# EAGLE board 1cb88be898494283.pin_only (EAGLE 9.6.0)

Size 43.18 x 43.18 mm. Coordinates in mm from the lower left corner, seen from the top.
Outline: 43.18,0 0,0 0,43.18 43.18,43.18 43.18,0
Copper layers (1+2*15+16): Top 0.035mm / dielectric 1.5mm / Route2 0.035mm / dielectric 0.15mm / Route15 0.035mm / dielectric 0.2mm / Bottom 0.035mm
Design rules "SparkFun-4-layer-MicroMod *": minimum track width 4mil, minimum drill 0.2mm, track to track 4mil, track to pad 4mil, pad to pad 4mil, via to via 4mil, smd to smd 4mil, copper to edge 6mil, drill to drill 6mil, minimum pad ring 6mil, minimum via ring 6mil, stop-mask expansion 4mil, vias tented up to drill 25mil, thermal gap 10mil
Net classes: 1 power: width 0.178 mm; 2 3.3V: width 0.508 mm; 3 RF: width 0.35 mm, clearance 0.203 mm

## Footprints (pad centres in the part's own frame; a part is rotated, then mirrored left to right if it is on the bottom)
ML414H_IV01E = smd 1 x 1: + 2.022,2.032 | smd 4.2 x 1.7: - 0.6,-1.85
0402 = smd 0.85 x 0.9: 1 -0.58,0; 2 0.58,0
0603 = smd 1.1 x 1: 1 -0.85,0; 2 0.85,0
LED-0603 = smd 1 x 1: A -0.877,0; C 0.877,0
SOD-323 = smd 0.63 x 0.83: A 1.15,0; C -1.15,0
SOT886 = smd 0.61 x 0.25: 1 -0.405,0.5 | smd 0.56 x 0.25: 2 -0.43,0; 3 -0.43,-0.5; 4 0.43,-0.5; 5 0.43,0; 6 0.43,0.5
SMA-EDGE = smd 1.5 x 4: GND@0 -2.54,0; GND@1 2.54,0; SIG 0,0 | smd 1.5 x 4 bottom: GND@2 -2.54,0; GND@3 2.54,0
0402_MURATA = smd 0.4 x 0.7: P1 -0.4,0; P2 0.4,0
SMT-JUMPER_2_NC_TRACE_SILK = smd 0.66 x 1.27: 1 -0.521,0; 2 0.521,0
1X06_NO_SILK = drill 1.016 pad 1.88: 1 0,0; 2 2.54,0; 3 5.08,0; 4 7.62,0; 5 10.16,0; 6 12.7,0
JST04_1MM_RA = smd 0.6 x 1.35: 1 -1.5,0; 2 -0.5,0; 3 0.5,0; 4 1.5,0 | smd 1.2 x 2: NC1 2.8,-3.675; NC2 -2.8,-3.675
1X04_NO_SILK = drill 1.016 pad 1.88: 1 0,0; 2 2.54,0; 3 5.08,0; 4 7.62,0
USB-C-16P-2LAYER-PADS = smd 0.3 x 1: A5 -1.25,-0.34; A6 -0.25,-0.34; A7 0.25,-0.34; A8 1.25,-0.34; B5 1.75,-0.34; B6 0.75,-0.34; B7 -0.75,-0.34; B8 -1.75,-0.34 | smd 0.6 x 1: GND -3.225,-0.34; GND2 3.225,-0.34; VBUS1 -2.45,-0.34; VBUS2 2.45,-0.34 | drill 0.4 pad 0.6 long: SHLD1 -4.318,-0.915; SHLD2 4.318,-0.915; SHLD3 -4.318,-5.095; SHLD4 4.318,-5.095 | hole 0.65: -2.89,-1.445; 2.89,-1.445
1X09_NO_SILK = drill 1.016 pad 1.88: 1 0,0; 2 2.54,0; 3 5.08,0; 4 7.62,0; 5 10.16,0; 6 12.7,0; 7 15.24,0; 8 17.78,0; 9 20.32,0
SMT-JUMPER_3_2-NC_TRACE_SILK = smd 0.66 x 1.27: 1 -1.041,0; 2 0,0; 3 1.041,0
MICRO-FIDUCIAL = smd 0.635 x 0.635: 1 0,0
STAND-OFF = hole 3.302: 0,0
SMT-JUMPER_2_NO_SILK = smd 0.635 x 1.27: 1 -0.406,0; 2 0.406,0
SOT23-5 = smd 0.55 x 1.2: 1 -0.95,-1.3; 2 0,-1.3; 3 0.95,-1.3; 4 0.95,1.3; 5 -0.95,1.3
ZED-F9P = smd 0.85 x 1.52: 1 -7.15,-7.45; 2 -6.05,-7.45; 3 -4.95,-7.45; 4 -3.85,-7.45; 5 -2.75,-7.45; 6 -1.65,-7.45; 7 -0.55,-7.45; 8 0.55,-7.45; 9 1.65,-7.45; 10 2.75,-7.45; 11 3.85,-7.45; 12 4.95,-7.45; 13 6.05,-7.45; 14 7.15,-7.45; 28 7.15,7.45; 29 6.05,7.45; 30 4.95,7.45; 31 3.85,7.45; 32 2.75,7.45; 33 1.65,7.45; 34 0.55,7.45; 35 -0.55,7.45; 36 -1.65,7.45; 37 -2.75,7.45; 38 -3.85,7.45; 39 -4.95,7.45; 40 -6.05,7.45; 41 -7.15,7.45 | smd 1.52 x 0.85: 15 9.95,-6.6; 16 9.95,-5.5; 17 9.95,-4.4; 18 9.95,-3.3; 19 9.95,-2.2; 20 9.95,-1.1; 21 9.95,0; 22 9.95,1.1; 23 9.95,2.2; 24 9.95,3.3; 25 9.95,4.4; 26 9.95,5.5; 27 9.95,6.6; 42 -9.95,6.6; 43 -9.95,5.5; 44 -9.95,4.4; 45 -9.95,3.3; 46 -9.95,2.2; 47 -9.95,1.1; 48 -9.95,0; 49 -9.95,-1.1; 50 -9.95,-2.2; 51 -9.95,-3.3; 52 -9.95,-4.4; 53 -9.95,-5.5; 54 -9.95,-6.6 | smd 1.1 x 1.1: 55 -1.05,-1.05; 56 -3.15,-1.05; 57 -5.25,-1.05; 58 -7.35,-1.05; 59 -1.05,-3.1; 60 -3.15,-3.1; 61 -5.25,-3.1; 62 -7.35,-3.1; 63 -1.05,-5.15; 64 -3.15,-5.15; 65 -5.25,-5.15; 66 -7.35,-5.15; 67 -1.05,5.15; 68 -3.15,5.15; 69 -5.25,5.15; 70 -7.35,5.15; 71 -1.05,3.1; 72 -3.15,3.1; 73 -5.25,3.1; 74 -7.35,3.1; 75 -1.05,1.05; 76 -3.15,1.05; 77 -5.25,1.05; 78 -7.35,1.05; 79 1.05,1.05; 80 3.15,1.05; 81 5.25,1.05; 82 7.35,1.05; 83 1.05,3.1; 84 3.15,3.1; 85 5.25,3.1; 86 7.35,3.1; 87 1.05,5.15; 88 3.15,5.15; 89 5.25,5.15; 90 7.35,5.15; 91 1.05,-5.15; 92 3.15,-5.15; 93 5.25,-5.15; 94 7.35,-5.15; 95 1.05,-3.1; 96 3.15,-3.1; 97 5.25,-3.1; 98 7.35,-3.1; 99 1.05,-1.05; 100 3.15,-1.05; 101 5.25,-1.05; 102 7.35,-1.05

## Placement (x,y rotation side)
B1  6.8MM_COIN_CELL  [ML414H_IV01E]  11.43,29.21 180 top
C1  47pF  [0402]  35.05,23.24 90 top
C2  1.0uF  [0603]  13.97,19.81 180 top
C3  1.0uF  [0603]  11.05,16.76 270 top
C4  1.0uF  [0603]  15.24,26.67 0 top
C5  0.1uF  [0603]  15.88,24.13 270 top
C6  1.0uF  [0603]  9.53,24.13 90 top
C7  0.1uF  [0603]  13.97,18.29 0 top
D1  Yellow  [LED-0603]  37.47,30.48 270 top
D2  0.5A/40V/420mV  [SOD-323]  13.97,21.34 0 top
D3  GREEN  [LED-0603]  39.37,30.48 270 top
D4  BLUE  [LED-0603]  41.27,30.48 270 top
D6  PRTR5V0U2F  [SOT886]  10.92,13.08 0 top
E1  SMA  [SMA-EDGE]  41.02,19.43 270 top
E2  SMA  [SMA-EDGE]  41.02,10.03 270 top
FB1  120NH  [0402_MURATA]  35.05,16.13 90 top
FENCE  [SMT-JUMPER_2_NC_TRACE_SILK]  41.27,31.75 270 bottom
FRAME2  FRAME-LEDGER  [CREATIVE_COMMONS]  not placed on the board
J1  Radio  [1X06_NO_SILK]  1.27,34.29 270 top
J2  Qwiic Right Angle  [JST04_1MM_RA]  8.89,5.08 0 top
J3  PTH  [1X04_NO_SILK]  13.97,1.27 0 top
J4  Qwiic Right Angle  [JST04_1MM_RA]  8.89,38.1 180 top
J5  [USB-C-16P-2LAYER-PADS]  6.35,12.7 270 top
J6  [1X06_NO_SILK]  24.13,1.27 0 top
J7  [1X09_NO_SILK]  34.29,41.91 180 top
JP5  [SMT-JUMPER_3_2-NC_TRACE_SILK]  11.43,8.89 0 top
JP21  FIDUCIALUFIDUCIAL  [MICRO-FIDUCIAL]  42.55,42.55 90 top
JP31  STAND-OFF  [STAND-OFF]  2.54,2.54 90 top
JP41  STAND-OFF  [STAND-OFF]  2.54,40.64 90 top
JP61  FIDUCIALUFIDUCIAL  [MICRO-FIDUCIAL]  0.64,0.64 90 top
JP71  FIDUCIALUFIDUCIAL  [MICRO-FIDUCIAL]  42.55,42.55 270 bottom
JP81  FIDUCIALUFIDUCIAL  [MICRO-FIDUCIAL]  0.64,0.64 270 bottom
JP91  STAND-OFF  [STAND-OFF]  40.64,2.54 90 top
JP101  STAND-OFF  [STAND-OFF]  40.64,40.64 90 top
LED2  RED  [LED-0603]  35.56,30.48 270 top
LOGO1  OSHW-LOGOMINI  [OSHW-LOGO-MINI]  2.54,5.59 0 bottom
LOGO2  SFE_LOGO_NAME_FLAME.1_INCH  [SFE_LOGO_NAME_FLAME_.1]  21.59,25.4 0 bottom
PPS  [SMT-JUMPER_2_NC_TRACE_SILK]  33.02,7.62 90 top
PPS_LED  [SMT-JUMPER_2_NC_TRACE_SILK]  36.2,31.75 270 bottom
PWR  [SMT-JUMPER_2_NC_TRACE_SILK]  33.78,31.75 270 bottom
R1  1k  [0603]  35.56,34.29 90 top
R2  33  [0603]  21.46,7.62 270 top
R3  33  [0603]  18.41,7.62 270 top
R4  33  [0603]  22.99,7.62 270 top
R5  1k  [0603]  10.92,20.32 90 top
R6  33  [0603]  19.94,7.62 270 top
R7  2.2k  [0603]  13.97,8.89 90 top
R8  2.2k  [0603]  8.89,8.89 90 top
R9  27  [0603]  13.97,13.72 0 top
R10  27  [0603]  13.97,15.24 0 top
R11  1k  [0603]  37.47,34.29 90 top
R12  1k  [0603]  39.37,34.29 90 top
R13  1k  [0603]  41.27,34.29 90 top
R14  33  [0603]  35.05,19.81 90 top
R15  100k  [0603]  13.97,16.76 0 top
R16  5.1k  [0603]  3.17,6.99 0 top
R17  5.1k  [0603]  3.17,18.41 0 top
R18  33  [0603]  29.72,7.62 270 top
R19  33  [0603]  26.67,7.62 270 top
R20  33  [0603]  28.19,7.62 270 top
R21  33  [0603]  31.24,7.62 270 top
R22  33  [0603]  20.45,35.56 90 top
R23  33  [0603]  18.92,35.56 90 top
R24  33  [0603]  26.42,35.56 90 top
R25  33  [0603]  27.94,35.56 90 top
RTK  [SMT-JUMPER_2_NC_TRACE_SILK]  38.73,31.75 270 bottom
SPI  [SMT-JUMPER_2_NO_SILK]  24.13,8.51 90 bottom
U2  3.3V  [SOT23-5]  12.7,24.13 270 top
U3  ZED-F9P  [ZED-F9P]  25.4,21.59 90 top
U$1  [SDA-[)]  19.05,1.65 90 top
U$2  SPECIAL_INSTRUCTIONS-ORDERING  [ORDERING_INSTRUCTIONS]  not placed on the board
U$3  [SCL-[)]  21.59,1.65 90 top
U$4  [SDA-[)]  19.05,1.65 90 bottom
U$5  [SCL-[)]  21.59,1.65 90 bottom
U$6  [3V3-04]  16.51,1.65 90 top
U$7  [3V3-04]  16.51,1.65 90 bottom
U$8  [GND-04]  13.97,1.65 90 top
U$9  [GND-04]  13.97,1.65 90 bottom
U$10  [I_SUPER2_C-()-03]  10.03,10.67 0 top
U$11  [FENCE2]  41.27,23.88 90 top
U$12  [PWR-()-03]  33.78,33.15 90 bottom
U$13  [RTK1]  39.37,25.27 90 top
U$14  [FENCE0]  24.13,1.78 90 top
U$15  [INT8]  36.83,1.65 90 top
U$16  [INT8]  36.83,1.65 90 bottom
U$17  [FENCE0]  24.13,1.78 90 bottom
U$18  [PWR-()-03]  35.56,25.02 90 top
U$19  [5V]  16.51,37.85 90 top
U$20  [5V]  16.51,37.85 90 bottom
U$21  [RX20]  24.13,36.83 90 top
U$22  [U#BLOX3]  26.16,22.61 0 bottom
U$23  [CS#-<]]  26.67,38.1 90 top
U$24  [CS#-<]]  26.67,38.1 90 bottom
U$25  [PPS0]  36.2,33.15 90 bottom
U$26  [RX#MOSI3]  29.21,34.42 90 top
U$27  [DSEL0]  26.16,10.54 0 bottom
U$28  [RTK1]  26.67,1.52 90 bottom
U$29  [RTK1]  26.67,1.52 90 top
U$30  [QWIIC_4MM]  8.89,6.6 0 top
U$31  [RX#MOSI3]  29.21,34.42 90 bottom
U$32  [RTK1]  38.73,33.15 90 bottom
U$33  [SFE_LOGO_FLAME_.1]  24,35.05 0 top
U$34  [TX#MISO1]  31.75,34.29 90 top
U$35  [#RST3]  31.75,1.4 90 top
U$36  [#RST3]  31.75,1.4 90 bottom
U$37  [TX#MISO1]  31.75,34.29 90 bottom
U$38  [SCK-(]-04]  34.29,37.08 90 top
U$39  [#SAFE1]  34.29,1.4 90 top
U$40  [#SAFE1]  34.29,1.4 90 bottom
U$41  [SCK-(]-04]  34.29,37.08 90 bottom
U$42  [RX22]  2.03,29.21 0 top
U$43  [PPS5]  29.21,1.65 90 top
U$44  [PPS5]  29.21,1.65 90 bottom
U$45  [GND3]  2.16,21.59 0 top
U$47  [PPS1]  38.1,8.26 90 top
U$48  [RTCM5]  6.73,37.85 0 bottom
U$49  [ZED#F9P6]  28.45,16.51 0 bottom
U$50  [TX21]  21.59,36.83 90 top
U$51  [TX23]  2.03,31.75 0 top
U$52  [PPS0]  37.47,25.4 90 top
U$53  [CORRECTION0]  8.89,36.58 0 bottom
U$54  [FENCE2]  41.27,33.15 90 bottom
U$55  [TX21]  21.59,36.83 90 bottom
U$56  [RX20]  24.13,36.83 90 bottom
U$57  [TX21]  6.86,31.75 0 bottom
U$58  [RX20]  6.73,29.21 0 bottom
U$59  [GPS0]  8,36.07 0 top
U$60  [3V3-04]  19.05,36.83 90 bottom
U$61  [3V3-04]  19.05,36.83 90 top
U$62  [GND-04]  13.97,36.7 90 bottom
U$63  [GND-04]  13.97,36.7 90 top
U$65  [ACTIVE_L1#L21]  38.1,15.49 90 top
U$66  [3V3-04]  2.03,26.67 0 top
U$67  [3V3-04]  6.73,26.67 0 bottom
U$68  [GND3]  6.99,21.59 0 bottom
U$69  [CORRECTION0]  -0.38,36.58 0 top
U$70  [RTCM5]  0.76,37.85 0 top
U$71  [ANTENNA2]  36.96,16.38 90 top
U$72  [PPS0]  34.29,7.75 0 top
U$73  [RTK#SMA4]  4.95,33.91 0 top
U$74  [PPS1]  38.1,11.81 270 bottom
U$75  [ANTENNA2]  38.1,22.35 270 bottom
U$76  [GPS#RTK#SMA5]  32.89,19.56 0 bottom

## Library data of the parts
B1 = SparkFun-Batteries; PROD_ID: BATT-14267
C1 = SparkFun-Capacitors; PROD_ID: CAP-15063
C2-C4 C6 = SparkFun-Capacitors; PROD_ID: CAP-13930
C5 C7 = SparkFun-Capacitors; PROD_ID: CAP-08604
D1 = SparkFun-LED; PROD_ID: DIO-09003
D2 = SparkFun-DiscreteSemi; PROD_ID: DIO-10955
D3 = SparkFun-LED; PROD_ID: DIO-00821
D4 = SparkFun-LED; PROD_ID: DIO-08575
D6 = SparkFun-IC-Power; PROD_ID: DIO-14084
E1 E2 = SparkFun-RF; PROD_ID: CONN-08289
FB1 = SparkFun-Coils; PROD_ID: NDUC-15072
FENCE JP5 PPS PPS_LED PWR RTK SPI = SparkFun-Jumpers
FRAME2 LOGO1 LOGO2 U$2 U$30 U$33 = SparkFun-Aesthetics
J1 J7 = SparkFun-Connectors
J2 J4 = SparkFun-Connectors; PROD_ID: CONN-13694
J3 = SparkX
J5 = SparkFun-Connectors; PROD_ID: CONN-14122
J6 = SparkFun-Connectors; PROD_ID: CONN-08437
JP21 JP31 JP41 JP61 JP71 JP81 JP91 JP101 = SparkFun
LED2 = SparkFun-LED; PROD_ID: DIO-00819
R1 R5 R11-R13 = SparkFun-Resistors; PROD_ID: RES-07856
R2-R4 R6 R14 R18-R25 = SparkFun-Resistors; PROD_ID: RES-08270
R7 R8 = SparkFun-Resistors; PROD_ID: RES-08272
R9 R10 = SparkFun-Resistors; PROD_ID: RES-09334
R15 = SparkFun-Resistors; PROD_ID: RES-07828
R16 R17 = SparkFun-Resistors; PROD_ID: RES-12083
U2 = SparkFun-IC-Power; PROD_ID: VREG-12457
U3 = ZED-F9P
U$1 U$3-U$10 U$12 U$18-U$20 U$23 U$24 U$38 U$41 U$60-U$63 U$66 U$67 = Labels
U$11 U$13 U$32 U$54 = buzzard_labels
U$14 U$17 U$28 U$29 = buzzard_labels (1)
U$15 U$16 U$22 = buzzard_labels (5)
U$21 U$42 U$50 U$51 U$55-U$58 = buzzard_labels (10)
U$25 U$52 U$72 = buzzard_labels (33)
U$26 U$31 U$34 U$37 = buzzard_labels (36)
U$27 = buzzard_labels (6)
U$35 U$36 U$39 U$40 U$43 U$44 = buzzard_labels (7)
U$45 U$48 U$49 U$53 U$59 U$68-U$70 U$76 = buzzard_labels (4)
U$47 U$74 = buzzard_labels (2)
U$65 U$71 U$75 = buzzard_labels (8)
U$73 = buzzard_labels (3)

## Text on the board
Bottom: v12-SMA
Measures: Measurements in inches
tDocu: Board thickness is 1.6mm | 4 Layer Board | No clean process

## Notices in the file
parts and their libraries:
SparkFun-Resistors: Licensing: Creative Commons ShareAlike 4.0 International - https://creativecommons.org/licenses/by-sa/4.0
SparkFun-Aesthetics: Released under the Creative Commons Attribution Share-Alike 4.0 License
SparkFun-Aesthetics: https://creativecommons.org/licenses/by-sa/4.0
